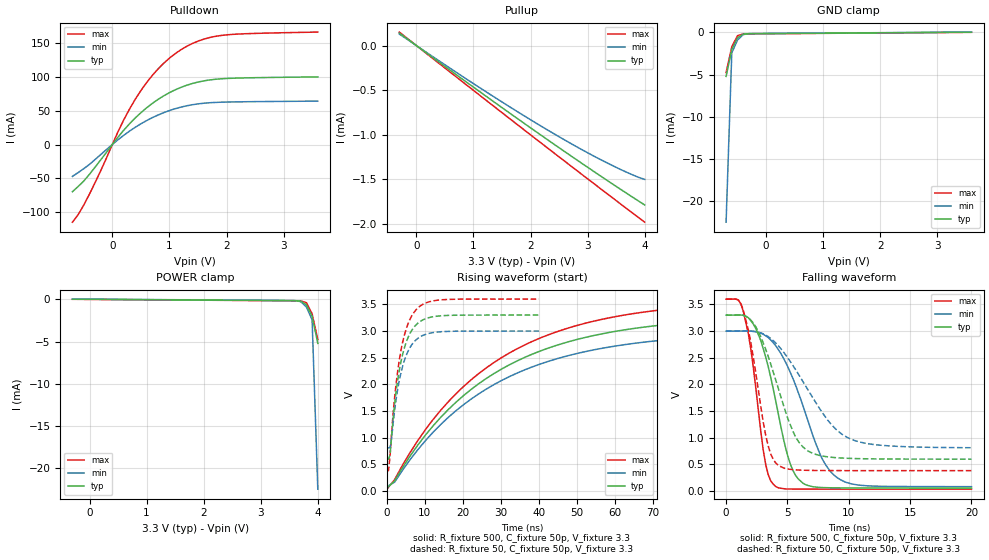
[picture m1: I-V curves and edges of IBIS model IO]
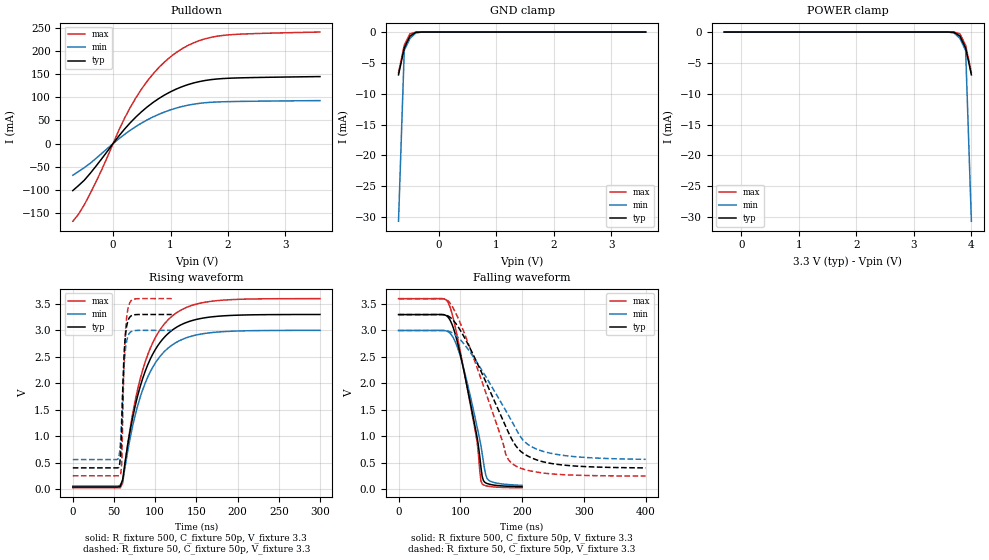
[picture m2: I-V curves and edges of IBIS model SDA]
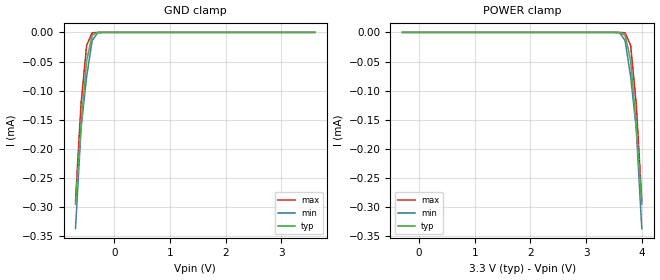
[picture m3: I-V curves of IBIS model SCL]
[IBIS Ver]   3.2
[Comment Char]   |_char
| VDD Nom: 3.3v, Min: 3v, Max: 3.6v
[File name]   pca9675_3_3v.ibs
[File Rev]   1
[Date]   08-25-2008
[Source]
[Notes]
[Disclaimer]
(C) Copyright 2007 NXP Semiconductors
All rights reserved
NXP Semiconductors (NXP) does not warrant that this model and any other
accompanying information (Model) accurately or fully represents the
operating characteristics and specifications of the semiconductor
products to which the Model relates.  Moreover, the Model is furnished
on an "as is" and with "all faults" basis, and without support or
warranty of any kind.  NXP disclaims all warranties, whether expressed
or implied or statutory, including without limitation all implied
warranties of non-infringement, merchantability and fitness for any
purpose, and those arising from a course of dealing or usage of trade.
NXP does not convey any license under its or any third party's patents,
copyrights or other intellectual property or proprietary rights.
You and your company assume any and all risks and liability arising out
of the application or use of the Model.
In no event shall NXP be liable for any direct, indirect, special,
consequential or incidental damages, however caused, whether in
warranty, contract or tort (including negligence), strict liability or
other legal theory, including, without limitation, for lost profits,
business interruption, or corruption or loss of data or information,
arising out of or in connection with the use of or the inability to use
the Model, even if NXP has been advised of the possibility of such
damages.
NXP provides the Model as a courtesy to our customers. You and your
company shall not distribute, convey, sell, or give the Model to anyone
else without receiving prior written permission from NXP.
NXP reserves the right to make changes without notice to the Model to
improve reliability, function, or design.
Please be aware that your receipt and subsequent use of the Model shall
serve as acceptance of these terms and conditions.  If you do not
accept these terms, return or destroy the Model immediately.
[Copyright]
2008
| SO24 package
[Component]   PCA9675D
Si_location Pin
Timing_location Pin
[Manufacturer]   NXP Semiconductors
[Package]
R_pkg   0.14   0.12   0.18
L_pkg   5.71n   3.95n   7.95n
C_pkg   1.01p   0.72p   1.49p
[Pin] signal_name   model_name   R_pin   L_pin   C_pin
1   INTb   INT   0.18   6.01n   0.97p
2   AD1   ADDR   0.14   7.94n   1.21p
3   AD2   ADDR   0.16   7.06n   1.32p
4   P00   IO   0.18   6.01n   1.07p
5   P01   IO   0.14   4.98n   0.88p
6   P02   IO   0.13   4.30n   0.80p
7   P03   IO   0.12   3.95n   0.74p
8   P04   IO   0.12   3.95n   0.72p
9   P05   IO   0.13   4.30n   0.76p
10   P06   IO   0.14   4.98n   0.85p
11   P07   IO   0.18   6.01n   0.97p
12   VSS   GND   0.16   7.06n   1.20p
13   P10   IO   0.14   7.95n   1.45p
14   P11   IO   0.14   7.95n   1.49p
15   P12   IO   0.16   7.06n   1.32p
16   P13   IO   0.18   6.01n   1.07p
17   P14   IO   0.14   4.98n   0.88p
18   P15   IO   0.13   4.30n   0.80p
19   P16   IO   0.12   3.95n   0.74p
20   P17   IO   0.12   3.95n   0.72p
21   AD0   ADDR   0.13   4.30n   0.76p
22   SCL   SCL   0.14   4.98n   0.85p
23   SDA   SDA   0.18   6.01n   0.97p
24   VDD   POWER   0.16   7.06n   1.20p
| TSSOP24 package
[Component]   PCA9675PW
Si_location Pin
Timing_location Pin
[Manufacturer]   NXP Semiconductors
[Package]
R_pkg   52.70m   31.50m   67.00m
L_pkg   2.19n   1.32n   3.39n
C_pkg   0.48p   0.35p   0.93p
[Pin] signal_name   model_name   R_pin   L_pin   C_pin
1   INTb   INT   66.40m   2.36n   0.47p
2   AD1   ADDR   66.10m   3.39n   0.57p
3   AD2   ADDR   67.00m   2.94n   0.59p
4   P00   IO   66.40m   2.36n   0.47p
5   P01   IO   47.10m   1.67n   0.40p
6   P02   IO   38.00m   1.44n   0.37p
7   P03   IO   31.50m   1.32n   0.35p
8   P04   IO   31.50m   1.32n   0.35p
9   P05   IO   38.00m   1.44n   0.37p
10   P06   IO   47.10m   1.67n   0.40p
11   P07   IO   66.40m   2.36n   0.47p
12   VSS   GND   67.00m   2.94n   0.59p
13   P10   IO   66.10m   3.39n   0.61p
14   P11   IO   66.20m   3.39n   0.61p
15   P12   IO   67.00m   2.94n   0.59p
16   P13   IO   66.50m   2.36n   0.47p
17   P14   IO   47.10m   1.67n   0.40p
18   P15   IO   38.00m   1.45n   0.37p
19   P16   IO   31.50m   1.32n   0.35p
20   P17   IO   31.50m   1.32n   0.35p
21   AD0   ADDR   38.00m   1.45n   0.37p
22   SCL   SCL   47.10m   1.67n   0.40p
23   SDA   SDA   66.50m   2.36n   0.47p
24   VDD   POWER   67.00m   2.94n   0.59p
| SSOP24
[Component]   PCA9675DB
Si_location Pin
Timing_location Pin
[Manufacturer]   NXP Semiconductors
[Package]
R_pkg   54.20m   39.70m   64.80m
L_pkg   2.55n   1.89n   3.58n
C_pkg   0.636p   0.52p   1.05p
[Pin] signal_name   model_name   R_pin   L_pin   C_pin
1   INTb   INT   63.00m   2.53n   0.58p
2   AD1   ADDR   61.20m   3.56n   0.70p
3   AD2   ADDR   64.80m   3.10n   0.76p
4   P00   IO   63.00m   2.53n   0.60p
5   P01   IO   52.60m   2.17n   0.57p
6   P02   IO   43.90m   2.03n   0.56p
7   P03   IO   39.70m   1.89n   0.54p
8   P04   IO   39.70m   1.89n   0.52p
9   P05   IO   43.90m   2.03n   0.55p
10   P06   IO   52.60m   2.17n   0.56p
11   P07   IO   63.00m   2.53n   0.58p
12   VSS   GND   64.80m   3.10n   0.71p
13   P10   IO   61.20m   3.56n   1.01p
14   P11   IO   61.20m   3.56n   1.05p
15   P12   IO   64.80m   3.10n   0.80p
16   P13   IO   63.00m   2.53n   0.65p
17   P14   IO   52.60m   2.17n   0.59p
18   P15   IO   43.90m   2.03n   0.56p
19   P16   IO   39.70m   1.89n   0.54p
20   P17   IO   39.70m   1.89n   0.53p
21   AD0   ADDR   43.90m   2.03n   0.56p
22   SCL   SCL   52.60m   2.17n   0.57p
23   SDA   SDA   63.00m   2.53n   0.60p
24   VDD   POWER   64.80m   3.10n   0.76p
[Define Package Model]  HVQFN24
[Manufacturer]  ST-NXP Wireless
|[Simulated] Chris Hunat
|[Approved] Wayne Nunn, Roger Real
[OEM]  Unknown
[Description]  Full package model
[Number Of Pins]  23
[Pin Numbers]
pin1   | pin1 = lead1
pin2   | pin2 = lead2
pin3   | pin3 = lead3
pin4   | pin4 = lead4
pin5   | pin5 = lead5
pin6   | pin6 = lead6
pin7   | pin7 = lead7
pin8   | pin8 = lead8
pin9   | pin9 = lead9
pin10   | pin10 = lead10
pin11   | pin11 = lead11
pin12   | pin12 = lead12
pin13   | pin13 = lead13
pin14   | pin14 = lead14
pin15   | pin15 = lead15
pin17   | pin17 = lead17
pin18   | pin18 = lead18
pin19   | pin19 = lead19
pin20   | pin20 = lead20
pin21   | pin21 = lead21
pin22   | pin22 = lead22
pin23   | pin23 = lead23
pin24   | pin24 = lead24
[Model Data]
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[End Model Data]
[End Package Model]
[Define Package Model]  DHVQFN24
[Manufacturer]  ST-NXP Wireless
|[Simulated] Chris Hunat
|[Approved] Wayne Nunn, Roger Real
[OEM]  Unknown
[Description]  Full package model
[Number Of Pins]  24
[Pin Numbers]
|Pin Num   Terminal Name
1   | lead1:pin1
2   | lead2:pin2
3   | lead3:pin3
4   | lead4:pin4
5   | lead5:pin5
6   | lead6:pin6
7   | lead7:pin7
8   | lead8:pin8
9   | lead9:pin9
10   | lead10:pin10
11   | lead11:pin11
12   | lead12:pin12
13   | lead13:pin13
14   | lead14:pin14
15   | lead15:pin15
16   | lead16:pin16
17   | lead17:pin17
18   | lead18:pin18
19   | lead19:pin19
20   | lead20:pin20
21   | lead21:pin21
22   | lead22:pin22
23   | lead23:pin23
24   | lead24:pin24
[Model Data]
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[End Model Data]
[End Package Model]
| Models and submodels in the file (5): IO (I/O), SDA (I/O_open_drain), SCL (Input), ADDR (Input), INT (Open_drain)
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[Model]   IO
Model_type I/O
Vinh=2.31
Vinl=0.99
Vref=3.3
Vmeas=1.65
Rref=500
Cref=50p
C_comp   7p   6.8p   7.2p
[Temperature Range] 27   85   -40
[Voltage Range]   3.3   3   3.6
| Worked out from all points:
|   slope of the pulldown table from 0 to 0.495 V, typ, clamps not added: 10.7 ohm
|   slope of the pullup table from 0 to 0.495 V, typ, clamps not added: 2.13 kohm
|   GND clamp passes 1 mA (typ) near -0.52 V on its own axis
|   falling waveform, R_fixture 500, C_fixture 50p, V_fixture 3.3: 20-80 % time 1.92ns typ, 2.86ns min, 1.18ns max; typ from 3.3 V to 0.059 V
|   falling waveform, R_fixture 50, C_fixture 50p, V_fixture 3.3: 20-80 % time 2.36ns typ, 3.75ns min, 1.38ns max; typ from 3.3 V to 0.6 V
|   rising waveform, R_fixture 500, C_fixture 50p, V_fixture 3.3: 20-80 % time 34.7ns typ, 34.9ns min, 34.6ns max; typ from 0.059 V to 3.3 V
|   rising waveform, R_fixture 50, C_fixture 50p, V_fixture 3.3: 20-80 % time 3.57ns typ, 3.59ns min, 3.56ns max; typ from 0.6 V to 3.3 V
[Pullup]
-300mV    140.2uA    129.3uA    150.8uA
1.1V      -512.3uA   -468.2uA   -552.5uA
2.3V      -1.056mA   -947uA     -1.149mA
2.8V      -1.277mA   -1.131mA   -1.395mA
3.3V      -1.493mA   -1.302mA   -1.64mA
3.7V      -1.662mA   -1.425mA   -1.835mA
4V        -1.787mA   -1.5mA     -1.98mA
[Pulldown]
-700mV    -69.7mA    -47.05mA   -114.6mA
-600mV    -61.98mA   -41.49mA   -103.5mA
-400mV    -43.82mA   -29.24mA   -72.96mA
-200mV    -22.2mA    -14.51mA   -37.9mA
100mV     11.05mA    7.118mA    19.12mA
400mV     39.11mA    25.38mA    66.64mA
700mV     60.68mA    39.63mA    102mA
900mV     71.84mA    47.03mA    119.9mA
1.1V      80.68mA    52.82mA    134.1mA
1.5V      92.18mA    59.98mA    152.6mA
1.9V      96.96mA    62.43mA    160.9mA
3.6V      99.8mA     64.04mA    165.9mA
[GND Clamp]
-700mV    -5.214mA   -22.45mA   -4.761mA
-600mV    -2.033mA   -2.422mA   -1.708mA
-500mV    -655.6uA   -909.6uA   -400.5uA
-400mV    -212.8uA   -276uA     -193uA
-200mV    -158.7uA   -141uA     -176.5uA
3.6V      13.62uA    27.33uA    109.1pA
[POWER Clamp]
-300mV    13.62uA    27.33uA    109.1pA
3.5V      -158.7uA   -141uA     -176.5uA
3.7V      -212.8uA   -276uA     -193uA
3.8V      -655.6uA   -909.6uA   -400.5uA
3.9V      -2.033mA   -2.422mA   -1.708mA
4V        -5.214mA   -22.45mA   -4.761mA
[Falling Waveform]
R_fixture=500
C_fixture=50p
V_fixture=3.3
V_fixture_min=3
V_fixture_max=3.6
0s        3.3V       3V         3.6V
1.414ns   3.296V     3.001V     3.361V
2.02ns    3.193V     2.999V     2.659V
3.232ns   2.511V     2.911V     495.3mV
4.04ns    1.695V     2.728V     86.12mV
5.051ns   638.1mV    2.321V     39.9mV
5.657ns   298.4mV    1.991V     38.06mV
7.677ns   68.69mV    681.9mV    36.84mV
9.091ns   61.17mV    246.7mV    36.7mV
20ns      58.61mV    83.38mV    36.65mV
[Falling Waveform]
R_fixture=50
C_fixture=50p
V_fixture=3.3
V_fixture_min=3
V_fixture_max=3.6
0s        3.3V       3V         3.6V
1.414ns   3.296V     3.001V     3.381V
2.02ns    3.204V     2.999V     2.782V
3.232ns   2.656V     2.923V     1.042V
4.242ns   1.936V     2.728V     485.7mV
5.455ns   1.12V      2.353V     402.8mV
6.263ns   829.5mV    2.054V     392.3mV
8.283ns   642.6mV    1.33V      385.4mV
9.899ns   615.3mV    1.004V     384.5mV
20ns      599.6mV    813.4mV    384.2mV
[Rising Waveform]
R_fixture=500
C_fixture=50p
V_fixture=3.3
V_fixture_min=3
V_fixture_max=3.6
0s        58.6mV     83.02mV    36.65mV
2.02ns    194.9mV    169.6mV    217.3mV
6.061ns   654.8mV    587mV      720.5mV
12.12ns   1.222V     1.102V     1.34V
22.22ns   1.909V     1.728V     2.09V
36.36ns   2.509V     2.275V     2.743V
52.53ns   2.886V     2.619V     3.152V
70.71ns   3.1V       2.816V     3.384V
96.97ns   3.23V      2.935V     3.525V
200ns     3.299V     2.999V     3.599V
[Rising Waveform]
R_fixture=50
C_fixture=50p
V_fixture=3.3
V_fixture_min=3
V_fixture_max=3.6
0s        599.5mV    809.9mV    384.2mV
404ps     599.5mV    809.9mV    384.5mV
808.1ps   675.1mV    817mV      657.9mV
1.212ns   1.027V     987.2mV    1.086V
2.02ns    1.637V     1.52V      1.763V
3.636ns   2.409V     2.202V     2.621V
5.253ns   2.827V     2.576V     3.081V
7.677ns   3.118V     2.836V     3.401V
14.14ns   3.286V     2.987V     3.584V
40ns      3.3V       3V         3.6V
[Ramp]
R_load=500
dV/dt_r   4.388E-2/1.281E-9   3.871E-2/1.430E-9   4.901E-2/1.040E-9
dV/dt_f   1.944E+0/5.484E-10   1.746E+0/9.304E-10   2.138E+0/2.734E-10
|[End   IO
| [End   SDA
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[Model]   SDA
Model_type I/O_open_drain
Vinh=2.31
Vinl=0.99
Vref=3.3
Vmeas=1.65
Rref=1k
Cref=50p
C_comp   6p   5.8p   6.2p
[Temperature Range] 27   85   -40
[Voltage Range]   3.3   3   3.6
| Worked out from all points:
|   slope of the pulldown table from 0 to 0.495 V, typ, clamps not added: 7.2 ohm
|   GND clamp passes 1 mA (typ) near -0.52 V on its own axis
|   falling waveform, R_fixture 500, C_fixture 50p, V_fixture 3.3: 20-80 % time 32.7ns typ, 33.2ns min, 33.5ns max; typ from 3.3 V to 0.051 V
|   falling waveform, R_fixture 50, C_fixture 50p, V_fixture 3.3: 20-80 % time 68.4ns typ, 73.8ns min, 60.6ns max; typ from 3.3 V to 0.407 V
|   rising waveform, R_fixture 500, C_fixture 50p, V_fixture 3.3: 20-80 % time 35.4ns typ, 35.5ns min, 35.3ns max; typ from 0.039 V to 3.3 V
|   rising waveform, R_fixture 50, C_fixture 50p, V_fixture 3.3: 20-80 % time 4.02ns typ, 4.65ns min, 3.77ns max; typ from 0.401 V to 3.3 V
[Pulldown]
-700mV    -101.5mA   -68.23mA   -167.9mA
-600mV    -90.64mA   -60.36mA   -152.5mA
-400mV    -64.71mA   -42.87mA   -108.7mA
-200mV    -33.19mA   -21.54mA   -57.19mA
200mV     31.35mA    19.98mA    54.76mA
400mV     57.83mA    37.18mA    99.59mA
700mV     89.28mA    57.92mA    151.2mA
1V        112.1mA    73.01mA    187.6mA
1.4V      131.1mA    85.2mA     217.8mA
1.8V      139.6mA    89.94mA    232mA
2.3V      142.4mA    91.39mA    237.1mA
3.6V      144.9mA    92.99mA    241.2mA
[GND Clamp]
-700mV    -6.935mA   -30.66mA   -6.593mA
-600mV    -2.591mA   -2.99mA    -2.148mA
-500mV    -653.7uA   -1.019mA   -278.6uA
-400mV    -54.45uA   -160.3uA   -7.607uA
-200mV    -25.65nA   -197.3nA   -667.7pA
3.6V      201.4pA    372.1pA    187.3pA
[POWER Clamp]
-300mV    201.4pA    372.1pA    187.3pA
3.5V      -25.65nA   -197.3nA   -667.7pA
3.7V      -54.45uA   -160.3uA   -7.607uA
3.8V      -653.7uA   -1.019mA   -278.6uA
3.9V      -2.591mA   -2.99mA    -2.148mA
4V        -6.935mA   -30.66mA   -6.593mA
[Falling Waveform]
R_fixture=500
C_fixture=50p
V_fixture=3.3
V_fixture_min=3
V_fixture_max=3.6
0s        3.3V       3V         3.6V
78.79ns   3.268V     2.984V     3.553V
88.89ns   3.042V     2.858V     3.215V
103ns     2.387V     2.39V      2.417V
125.3ns   1.101V     1.282V     1.034V
133.3ns   426.1mV    826.3mV    164.6mV
135.4ns   250.7mV    681.8mV    104.8mV
141.4ns   122.1mV    264.8mV    70.15mV
145.5ns   104.2mV    177.8mV    60.03mV
200ns     51.46mV    77.03mV    30.61mV
[Falling Waveform]
R_fixture=50
C_fixture=50p
V_fixture=3.3
V_fixture_min=3
V_fixture_max=3.6
0s        3.3V       3V         3.6V
72.73ns   3.298V     2.999V     3.599V
84.85ns   3.236V     2.968V     3.493V
117.2ns   2.631V     2.57V      2.621V
165.7ns   1.395V     1.647V     998.2mV
173.7ns   1.183V     1.485V     656.7mV
185.9ns   894.7mV    1.234V     471.4mV
206.1ns   650.9mV    879.2mV    369.6mV
238.4ns   510.1mV    704.7mV    304.2mV
400ns     407mV      568.6mV    252.9mV
[Rising Waveform]
R_fixture=500
C_fixture=50p
V_fixture=3.3
V_fixture_min=3
V_fixture_max=3.6
0s        39.15mV    56.18mV    24.11mV
57.58ns   50.17mV    74.27mV    23.92mV
60.61ns   185.4mV    154.2mV    117.1mV
66.67ns   839.7mV    719.9mV    851.4mV
75.76ns   1.576V     1.401V     1.675V
87.88ns   2.228V     2.004V     2.405V
103ns     2.708V     2.45V      2.941V
124.2ns   3.043V     2.76V      3.314V
172.7ns   3.262V     2.964V     3.558V
300ns     3.3V       3V         3.6V
[Rising Waveform]
R_fixture=50
C_fixture=50p
V_fixture=3.3
V_fixture_min=3
V_fixture_max=3.6
0s        401.2mV    558.1mV    250.6mV
53.33ns   401.2mV    558mV      250.6mV
56.97ns   478.9mV    709.5mV    250.6mV
58.18ns   677.9mV    958mV      284.5mV
59.39ns   1.179V     1.364V     476.7mV
61.82ns   2.406V     2.209V     2.2V
63.03ns   2.746V     2.501V     2.727V
65.45ns   3.086V     2.806V     3.263V
67.88ns   3.218V     2.925V     3.471V
120ns     3.3V       3V         3.6V
[Ramp]
R_load=500
dV/dt_r   1.957E+0/1.366E-9   1.943E+0/1.981E-9   1.967E+0/8.995E-10
dV/dt_f   1.956E+0/3.194E-8   1.942E+0/3.578E-8   1.967E+0/2.977E-8
|[End   SDA
| [End   SCL
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[Model]   SCL
Model_type Input
Vinh=2.31
Vinl=0.99
C_comp   5p   4.8p   5.2p
[Temperature Range] 27   85   -40
[Voltage Range]   3.3   3   3.6
[GND Clamp]
-700mV    -295uA     -337uA     -289.5uA
-600mV    -158.8uA   -164.3uA   -122uA
-500mV    -48.62uA   -75.94uA   -22.35uA
-400mV    -4.926uA   -13.83uA   -710.6nA
-300mV    -138.4nA   -722.3nA   -7.551nA
3.6V      8.544pA    24.57pA    7.213pA
[POWER Clamp]
-300mV    8.544pA    24.57pA    7.213pA
3.6V      -138.4nA   -722.3nA   -7.551nA
3.7V      -4.926uA   -13.83uA   -710.6nA
3.8V      -48.62uA   -75.94uA   -22.35uA
3.9V      -158.8uA   -164.3uA   -122uA
4V        -295uA     -337uA     -289.5uA
